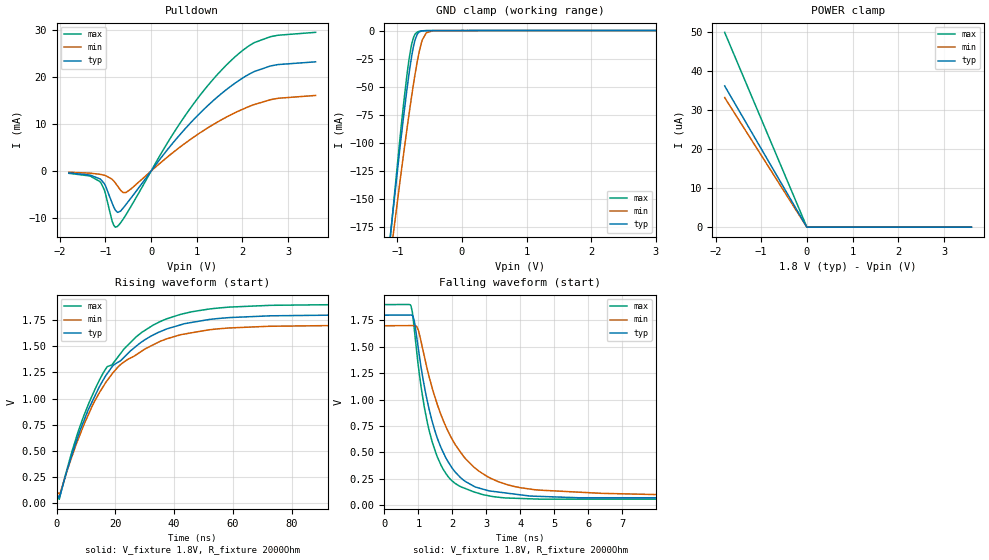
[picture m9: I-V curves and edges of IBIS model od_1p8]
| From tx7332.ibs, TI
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|   od_1p8 Model
[Model]   od_1p8
Model_type   Open_drain
Polarity   Inverting
Vmeas = 0.9
Vref = 1.8
Cref = 2pF
Rref = 2000
|   typ   min   max
C_comp   6.602pF   6.602pF   6.663pF
| Where Nom  PVT is Nominal Process, 1.8V, 27C
|   Fast PVT is Strong Process,  1.9V, 0C
|   Slow PVT is Weak Process,   1.7V, 100C
[Voltage Range]   1.8   1.7   1.9
|Junction Temperature
[Temperature Range]   27   100   0
[Pullup Reference]   1.8   1.7   1.9
[Pulldown Reference]   0   0   0
[Power Clamp Reference]   1.8   1.7   1.9
[GND Clamp Reference]   0   0   0
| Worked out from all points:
|   slope of the pulldown table from 0 to 0.27 V, typ, clamps not added: 77.8 ohm
|   GND clamp passes 1 mA (typ) near -0.65 V on its own axis
|   falling waveform, V_fixture 1.8V, R_fixture 2000Ohm: 20-80 % time 858ps typ, 1.26ns min, 679ps max; typ from 1.8 V to 0.068 V
|   rising waveform, V_fixture 1.8V, R_fixture 2000Ohm: 20-80 % time 20.4ns typ, 19.7ns min, 20.4ns max; typ from 0.068 V to 1.8 V
[Pulldown]
|   Voltage   I(typ)   I(min)   I(max)
-1.8V     -409.9uA   -254.5uA   -481.4uA
-1.341V   -844.5uA   -446uA     -1.041mA
-1.12V    -1.664mA   -689.1uA   -2.242mA
-1.017V   -2.809mA   -913.1uA   -4.223mA
-849.6mV  -6.902mA   -1.781mA   -10.74mA
-736.2mV  -8.775mA   -3.161mA   -11.78mA
-547.2mV  -7.081mA   -4.557mA   -9.252mA
662.4mV   8.085mA    5.319mA    10.61mA
1.688V    17.63mA    11.68mA    22.94mA
2.142V    20.59mA    13.72mA    26.64mA
2.612V    22.35mA    15.17mA    28.58mA
3.6V      23.24mA    16.08mA    29.51mA
[GND Clamp]
|   Voltage   I(typ)   I(min)   I(max)
-1.8V     -566.2mA   -530.2mA   -621.2mA
-1.13V    -194.2mA   -212.3mA   -197.4mA
-963mV    -106.3mA   -136.2mA   -98.01mA
-898.2mV  -74.21mA   -107.8mA   -62.58mA
-822.6mV  -39.93mA   -75.95mA   -27.03mA
-784.8mV  -25.18mA   -60.8mA    -13.99mA
-752.4mV  -14.76mA   -48.43mA   -6.624mA
-693mV    -3.429mA   -27.96mA   -1.353mA
-612mV    -259.3uA   -8.159mA   -259.6uA
-552.6mV  -71.87uA   -2.025mA   -111.7uA
-444.6mV  -45.53uA   -126.1uA   -66.75uA
3.6V      0A         0A         0A
[POWER Clamp]
|   Voltage   I(typ)   I(min)   I(max)
-1.8V     36.14uA    33.16uA    49.83uA
-7.2mV    108.4nA    96.74nA    163.4nA
-1.8mV    54.2nA     48.37nA    13.88nA
3.6V      0A         0A         0A
[Ramp]
R_load = 2000
|   typ   min   max
dV/dt_r   1.03907/2.03882e-08   0.962161/1.96575e-08   1.10655/2.02942e-08
dV/dt_f   1.03907/8.57406e-10   0.962161/1.25993e-09   1.10655/6.76712e-10
[Falling Waveform]
V_fixture = 1.8V
V_fixture_min = 1.7V
V_fixture_max = 1.9V
R_fixture = 2000Ohm
C_fixture = 0F
|   Time   V(typ)   V(min)   V(max)
0s        1.8V       1.7V       1.9V
782.1ps   1.801V     1.701V     1.888V
876.5ps   1.75V      1.701V     1.675V
1ns       1.478V     1.655V     1.314V
1.263ns   986.4mV    1.285V     782.9mV
1.526ns   664.9mV    985.2mV    483.8mV
1.854ns   422.6mV    714.1mV    280mV
2.987ns   144.4mV    279.8mV    94.76mV
4.56ns    83.72mV    143mV      57.67mV
300ns     68.21mV    96.39mV    55.74mV
[Rising Waveform]
V_fixture = 1.8V
V_fixture_min = 1.7V
V_fixture_max = 1.9V
R_fixture = 2000Ohm
C_fixture = 0F
|   Time   V(typ)   V(min)   V(max)
0s        68.21mV    96.39mV    55.74mV
923.5ps   54.83mV    90.58mV    36.89mV
5.114ns   452mV      435.1mV    480.9mV
9.058ns   769.6mV    732.5mV    819.2mV
17.04ns   1.231V     1.165V     1.297V
22.14ns   1.372V     1.334V     1.444V
29.12ns   1.545V     1.457V     1.636V
46.17ns   1.729V     1.631V     1.831V
95.42ns   1.799V     1.699V     1.899V
300ns     1.8V       1.7V       1.9V
